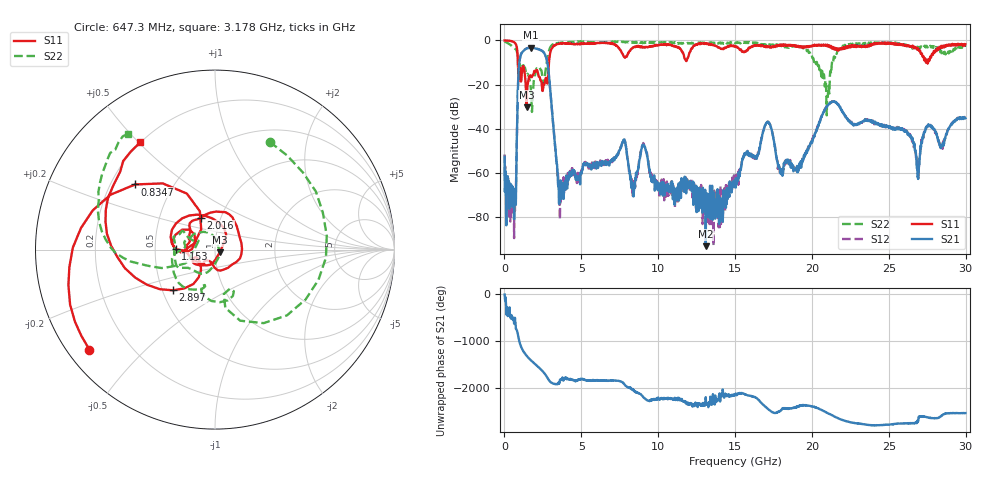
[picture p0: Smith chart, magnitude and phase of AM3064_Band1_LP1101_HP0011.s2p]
# Hz S DB R 50.0
!freq dBS11 angS11 dBS21 angS21 dBS12 angS12 dBS22 angS22
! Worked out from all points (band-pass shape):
!   1600 points, 10 MHz to 29.98 GHz, reference 50 ohm
!   highest |S21| = -3.29 dB at 1.716 GHz (marker M1); lowest = -93.1 dB at 13.09 GHz (marker M2)
!   |S21| within 3 dB of the highest: 1.077 GHz to 2.628 GHz (1.551 GHz wide, 83.7 % of centre)
!   lowest |S11| = -30.3 dB at 1.435 GHz (marker M3), VSWR 1.06, Z = 52.7 - j1.6 ohm
!   |S11| at or under -10 dB: 876.7 MHz to 2.893 GHz (2.016 GHz wide, 107 % of centre); 27.4193 GHz to 27.43556 GHz (16.26 MHz wide, 0.0593 % of centre); 27.51032 GHz to 27.55284 GHz (42.52 MHz wide, 0.154 % of centre)
!   |S22| runs from -33.9 to -0.4 dB; largest |S21 - S12| = 0.0096
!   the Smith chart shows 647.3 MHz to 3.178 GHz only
!   S11 on the Smith chart (normalised r, x): 647.3 MHz: 0.06, -0.35; 834.7 MHz: 0.30, +0.33; 1.153 GHz: 0.64, +0.00; 2.016 GHz: 0.81, +0.30; 2.897 GHz: 0.57, -0.29; 3.178 GHz: 0.20, +0.50
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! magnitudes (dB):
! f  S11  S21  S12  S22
! 10 MHz  0.0  -52.7  -51.6  -0.4
! 647.3 MHz  -1.0  -70.1  -68.0  -3.4
! 834.7 MHz  -4.8  -34.1  -34.0  -6.2
! 1.153 GHz  -13.2  -5.4  -5.3  -12.4
! 1.435 GHz  -30.3  -3.7  -3.6  -15.5
! 1.716 GHz  -16.0  -3.3  -3.3  -21.9
! 2.016 GHz  -14.3  -3.6  -3.5  -14.8
! 2.897 GHz  -9.7  -16.0  -15.9  -4.7
! 3.178 GHz  -2.8  -38.7  -38.6  -1.9
! 3.628 GHz  -1.4  -71.9  -69.8  -1.1
! 5.015 GHz  -1.5  -60.3  -58.5  -0.6
! 7.751 GHz  -7.2  -45.2  -45.1  -0.6
! 10 GHz  -2.1  -67.3  -65.1  -0.9
! 13.09 GHz  -1.5  -93.1  -76.7  -0.9
! 15 GHz  -2.8  -64.6  -65.0  -1.3
! 17.09 GHz  -2.6  -36.9  -37.0  -2.0
! 18 GHz  -2.0  -58.4  -60.5  -2.6
! 19.99 GHz  -2.7  -45.6  -45.3  -6.9
! 20.98 GHz  -2.2  -30.0  -29.6  -26.3
! 25 GHz  -1.1  -39.6  -38.8  -1.2
! 26.89 GHz  -3.9  -61.5  -58.2  -3.2
! 29.98 GHz  -1.8  -35.2  -35.1  -2.9
